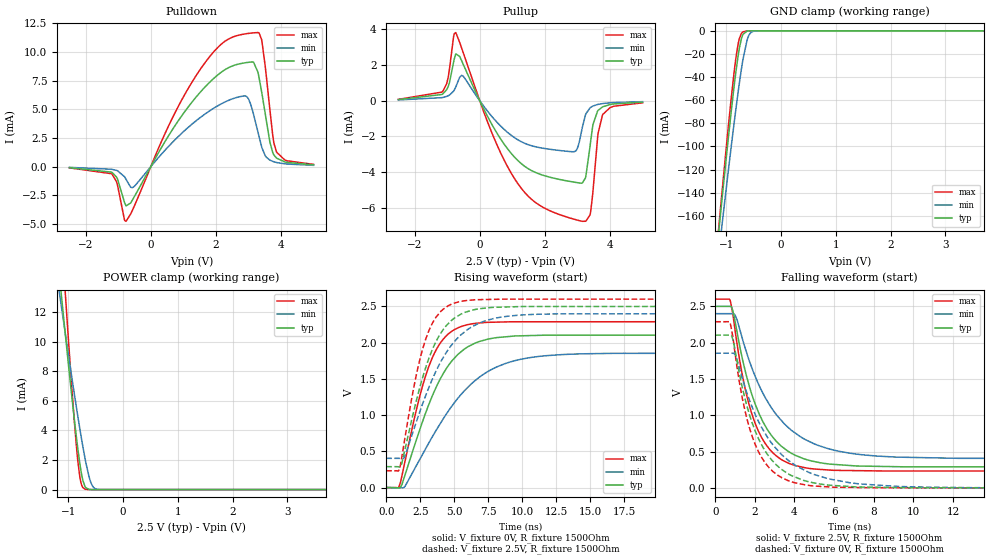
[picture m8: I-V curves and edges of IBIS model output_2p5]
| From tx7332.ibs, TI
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|   output_2p5 Model
[Model]   output_2p5
Model_type   3-state
Polarity   Non-Inverting
Vmeas = 1.25
Vref = 0
Cref = 2pF
Rref = 100000
|   typ   min   max
C_comp   5.803pF   5.724pF   5.857pF
| Where Nom  PVT is Nominal Process, 2.5V, 27C
|   Fast PVT is Strong Process,  2.6V, 0C
|   Slow PVT is Weak Process,   2.4V, 100C
[Voltage Range]   2.5   2.4   2.6
|Junction Temperature
[Temperature Range]   27   100   0
[Pullup Reference]   2.5   2.4   2.6
[Pulldown Reference]   0   0   0
[Power Clamp Reference]   2.5   2.4   2.6
[GND Clamp Reference]   0   0   0
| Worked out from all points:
|   slope of the pulldown table from 0 to 0.375 V, typ, clamps not added: 198 ohm
|   slope of the pullup table from 0 to 0.375 V, typ, clamps not added: 281 ohm
|   GND clamp passes 1 mA (typ) near -0.64 V on its own axis
|   POWER clamp passes 1 mA (typ) near -0.75 V on its own axis
|   falling waveform, V_fixture 2.5V, R_fixture 1500Ohm: 20-80 % time 1.65ns typ, 2.38ns min, 1.29ns max; typ from 2.5 V to 0.288 V
|   rising waveform, V_fixture 0V, R_fixture 1500Ohm: 20-80 % time 2.77ns typ, 4.17ns min, 2ns max; typ from 0 V to 2.1 V
|   rising waveform, V_fixture 2.5V, R_fixture 1500Ohm: 20-80 % time 2.16ns typ, 2.92ns min, 1.66ns max; typ from 0.288 V to 2.5 V
|   falling waveform, V_fixture 0V, R_fixture 1500Ohm: 20-80 % time 1.6ns typ, 2.33ns min, 1.25ns max; typ from 2.1 V to 0 V
[Pulldown]
|   Voltage   I(typ)   I(min)   I(max)
-2.5V     -89.37uA   -59.67uA   -103.3uA
-1.188V   -509.9uA   -233.3uA   -663.3uA
-760mV    -3.422mA   -1.108mA   -4.766mA
-512.5mV  -2.649mA   -1.733mA   -3.476mA
642.5mV   3.133mA    2.055mA    4.123mA
1.587V    6.713mA    4.431mA    8.765mA
2.908V    9.069mA    6.167mA    11.59mA
3.29V     8.263mA    3.053mA    11.7mA
3.417V    6.33mA     1.62mA     10.87mA
3.658V    2.163mA    575.4uA    5.006mA
3.86V     759.4uA    366.5uA    1.304mA
5V        159.4uA    116.6uA    200.6uA
[GND Clamp]
|   Voltage   I(typ)   I(min)   I(max)
-2.5V     -848.7mA   -784.5mA   -902.1mA
-1.165V   -187.9mA   -205.2mA   -185.3mA
-1.075V   -145.4mA   -167.7mA   -139.2mA
-1.067V   -141.9mA   -164.6mA   -135.5mA
-902.5mV  -67.67mA   -98.18mA   -56.03mA
-820mV    -34.66mA   -66.83mA   -22.83mA
-760mV    -15.26mA   -45.58mA   -6.838mA
-692.5mV  -3.035mA   -24.52mA   -855.5uA
-595mV    -102.3uA   -4.889mA   -53.23uA
-542.5mV  -14.91uA   -1.29mA    -12.69uA
-467.5mV  -897.5nA   -147.3uA   -1.327uA
5V        0A         0A         0A
[Pullup]
|   Voltage   I(typ)   I(min)   I(max)
-2.5V     66.87uA    45.76uA    81.89uA
-1.127V   396uA      187.9uA    556.5uA
-737.5mV  2.629mA    772.9uA    3.821mA
-512.5mV  2.059mA    1.381mA    2.714mA
387.5mV   -1.377mA   -915.1uA   -1.869mA
1.153V    -3.317mA   -2.168mA   -4.597mA
2.9V      -4.56mA    -2.853mA   -6.638mA
3.147V    -4.614mA   -1.514mA   -6.754mA
3.395V    -2.432mA   -386.3uA   -6.327mA
3.635V    -535.7uA   -201.8uA   -1.818mA
3.77V     -344.1uA   -158uA     -792.7uA
5V        -76.16uA   -50.31uA   -114.2uA
[POWER Clamp]
|   Voltage   I(typ)   I(min)   I(max)
-2.5V     65.02mA    47.85mA    97.77mA
-1.225V   16.9mA     14.98mA    23.12mA
-1.075V   11.34mA    11.14mA    14.55mA
-1.067V   11.07mA    10.95mA    14.13mA
-992.5mV  8.369mA    9.064mA    10mA
-887.5mV  4.761mA    6.479mA    4.634mA
-820mV    2.664mA    4.876mA    1.82mA
-760mV    1.142mA    3.516mA    382.1uA
-692.5mV  207.4uA    2.111mA    27.66uA
-580mV    3.225uA    427.6uA    200.6nA
-452.5mV  0A         12.92uA    0A
5V        0A         0A         0A
[Ramp]
R_load = 1500
|   typ   min   max
dV/dt_r   1.26271/2.76619e-09   1.11279/4.17084e-09   1.37322/1.99754e-09
dV/dt_f   1.32704/1.65315e-09   1.19797/2.37917e-09   1.42085/1.29249e-09
[Falling Waveform]
V_fixture = 2.5V
V_fixture_min = 2.4V
V_fixture_max = 2.6V
R_fixture = 1500Ohm
C_fixture = 0F
|   Time   V(typ)   V(min)   V(max)
0s        2.5V       2.4V       2.6V
749.9ps   2.5V       2.4V       2.586V
1ns       2.3V       2.383V     2.177V
1.498ns   1.631V     1.939V     1.383V
1.841ns   1.293V     1.66V      1.025V
2.342ns   948.1mV    1.338V     692.6mV
3.318ns   578.4mV    935mV      394.5mV
4.552ns   394.1mV    664.5mV    275.9mV
9.134ns   291.8mV    423.8mV    232.5mV
50ns      288.3mV    403.4mV    231.9mV
[Rising Waveform]
V_fixture = 0V
V_fixture_min = 0V
V_fixture_max = 0V
R_fixture = 1500Ohm
C_fixture = 0F
|   Time   V(typ)   V(min)   V(max)
0s        -858.1pV   603nV      -250.1nV
950.8ps   -3.221mV   -2.756mV   18.44mV
1.38ns    171.6mV    15.59mV    358.9mV
2.523ns   828.2mV    407mV      1.3V
3.533ns   1.326V     745.9mV    1.849V
4.552ns   1.678V     1.051V     2.117V
5.983ns   1.94V      1.379V     2.248V
8.794ns   2.08V      1.714V     2.286V
12.94ns   2.102V     1.835V     2.288V
50ns      2.105V     1.855V     2.289V
[Rising Waveform]
V_fixture = 2.5V
V_fixture_min = 2.4V
V_fixture_max = 2.6V
R_fixture = 1500Ohm
C_fixture = 0F
|   Time   V(typ)   V(min)   V(max)
0s        288.3mV    403.4mV    231.9mV
1.026ns   289.2mV    402.4mV    295.4mV
1.362ns   511.5mV    424.1mV    666.2mV
2.17ns    1.162V     880.8mV    1.514V
3.145ns   1.785V     1.383V     2.167V
4.245ns   2.194V     1.811V     2.468V
5.341ns   2.376V     2.079V     2.563V
7.306ns   2.477V     2.302V     2.595V
11.2ns    2.498V     2.392V     2.599V
50ns      2.5V       2.4V       2.6V
[Falling Waveform]
|Gnd
V_fixture = 0V
V_fixture_min = 0V
V_fixture_max = 0V
R_fixture = 1500Ohm
C_fixture = 0F
|   Time   V(typ)   V(min)   V(max)
0s        2.105V     1.855V     2.289V
749.9ps   2.105V     1.855V     2.275V
1.046ns   1.83V      1.813V     1.767V
1.498ns   1.237V     1.394V     1.068V
2.342ns   593.7mV    831.9mV    417.9mV
3.318ns   259.8mV    467.7mV    146.8mV
4.552ns   95.9mV     237.2mV    40.15mV
6.774ns   18.76mV    71.24mV    6.293mV
10.72ns   1.117mV    9.241mV    500.3uV
50ns      -54nV      200.1nV    -263.5nV
